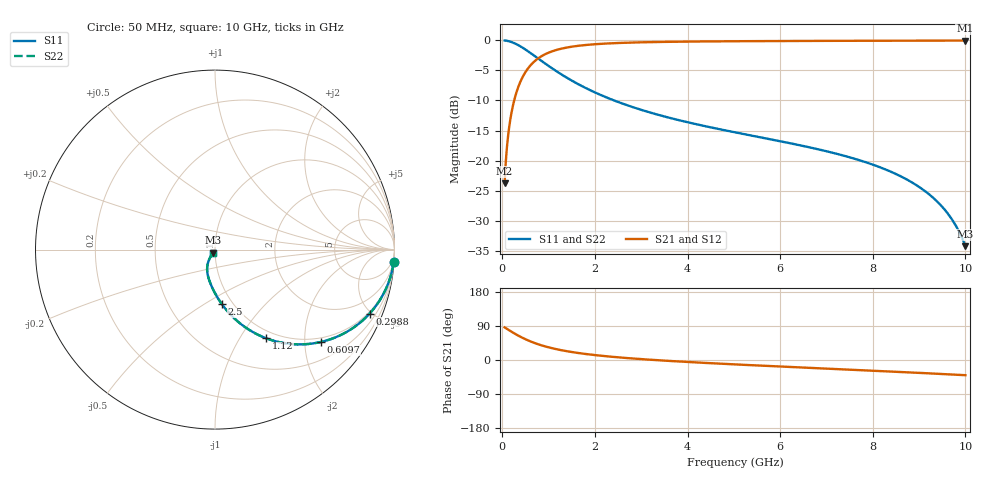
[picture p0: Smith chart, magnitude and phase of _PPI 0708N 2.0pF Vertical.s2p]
! S-Parameter data specifications (vertical orientation):
! Substrate: 40-mil Rogers 3003C, Substrate thickness, H=1.016mm, Dielectric constant, Er=3, Conductor thickness, T_mtl=0.043mm, Loss Tangent, Tand=0.003
! PCB Mounting Pad Footprint: Pad width, PadW=2.54mm , Pad length, PadL=0.51mm , Pad gap, PadG (edge-to-edge)=0.71mm , Reference planes=1.73mm apart
! Created Tue Jan 16 08:44:12 2018
# GHz S MA R 50
! 2 Port Network Data from SP1.SP block
! freq  magS11  angS11  magS21  angS21  magS12  angS12  magS22  angS22
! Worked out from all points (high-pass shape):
!   801 points, 50 MHz to 10 GHz, reference 50 ohm
!   highest |S21| = -0.04 dB at 9.988 GHz (marker M1); lowest = -23.8 dB at 50 MHz (marker M2)
!   |S21| within 3 dB of the highest: 767.9 MHz to end of sweep
!   lowest |S11| = -34.2 dB at 10 GHz (marker M3), VSWR 1.04, Z = 49.1 - j1.68 ohm
!   |S11| at or under -10 dB: 2.415 GHz to end of sweep
!   |S22| runs from -34.2 to 0.0 dB; largest |S21 - S12| = 0
!   S11 on the Smith chart (normalised r, x): 50 MHz: 1, -29; 298.8 MHz: 0.89, -4.86; 609.7 MHz: 0.89, -2.39; 1.12 GHz: 0.89, -1.31; 2.5 GHz: 0.89, -0.60; 10 GHz: 0.98, -0.03
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0.05  0.9979 -3.9  0.06493 86.1  0.06493 86.1  0.9979 -3.9
0.124625  0.9871 -9.8  0.1601 80.2  0.1601 80.2  0.9871 -9.8
0.1619375  0.9785 -12.6  0.2062 77.4  0.2062 77.4  0.9785 -12.6
0.224125  0.96 -17.2  0.2799 72.8  0.2799 72.8  0.96 -17.2
0.29875  0.9321 -22.5  0.3621 67.5  0.3621 67.5  0.9321 -22.5
0.4355625  0.8702 -31.4  0.4924 58.6  0.4924 58.6  0.8702 -31.4
0.6096875  0.7842 -41.0  0.6201 49.0  0.6201 49.0  0.7842 -41.0
0.8584375  0.6691 -51.7  0.7425 38.3  0.7425 38.3  0.6691 -51.7
1.119625  0.5698 -60.1  0.821 29.9  0.821 29.9  0.5698 -60.1
1.39325  0.4889 -66.7  0.8714 23.2  0.8714 23.2  0.4889 -66.7
1.716625  0.4169 -72.7  0.9079 17.2  0.9079 17.2  0.4169 -72.7
2.500188  0.3073 -82.7  0.9504 7.1  0.9504 7.1  0.3073 -82.7
3.370812  0.2401 -90.3  0.9692 -0.7  0.9692 -0.7  0.2401 -90.3
5.025  0.1718 -101.0  0.9831 -11.6  0.9831 -11.6  0.1718 -101.0
6.691625  0.1274 -110.0  0.9893 -21.0  0.9893 -21.0  0.1274 -110.0
7.624437  0.1031 -114.7  0.9917 -26.1  0.9917 -26.1  0.1031 -114.7
8.345812  0.08221 -118.1  0.9933 -30.2  0.9933 -30.2  0.08221 -118.1
8.917938  0.06333 -120.5  0.9944 -33.5  0.9944 -33.5  0.06333 -120.5
9.365687  0.04664 -121.8  0.995 -36.1  0.995 -36.1  0.04664 -121.8
9.713938  0.03225 -121.5  0.9953 -38.3  0.9953 -38.3  0.03225 -121.5
9.987562  0.01999 -118.3  0.9954 -40.0  0.9954 -40.0  0.01999 -118.3
10  0.01942 -118.0  0.9954 -40.1  0.9954 -40.1  0.01942 -118.0
